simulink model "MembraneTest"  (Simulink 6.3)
settings: Solver=ode45  StartTime=0.0  StopTime=SimTime  FixedStep=0.001  RelTol=1e-3
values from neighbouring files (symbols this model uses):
  b = S/Sm    (= 0.1)    [Constantes.m]    (also in ConstantesBck.m)
  C = 1    [Constantes.m]    (also in ConstantesBck.m)
  Fact = 10^2    (= 100)    [Constantes.m]    (also in ConstantesBck.m)
  FreqStim = 1/(2*pi*i)    [SinPureTest.m]    (also in SinPureTestFreq.m; HalfSin.m; ScriptFour.m = 0.318309886184)
  gk = 36    [Constantes.m]    (also in ConstantesBck.m; sim_hh.m)
  gl = 0.3    [Constantes.m]    (also in ConstantesBck.m; sim_hh.m)
  gna = 120    [Constantes.m]    (also in ConstantesBck.m; sim_hh.m)
  h0 = 0.5961    [Constantes.m]    (also in ConstantesBck.m)
  IStim1 = AddI    (= 0)    [SinPureTest.m]    (also in SinPureTestFreq.m; ouin.m = -3000; TestStim.m; BiPhTest.m)
  m0 = 0.0529    [Constantes.m]    (also in ConstantesBck.m)
  mK = 0    [Constantes.m]    (also in ConstantesBck.m)
  mL = 0    [Constantes.m]    (also in ConstantesBck.m)
  mNa = 0    [Constantes.m]    (also in ConstantesBck.m)
  n0 = 0.3177    [Constantes.m]    (also in ConstantesBck.m)
  PhaseStim = 0    [SinPureTest.m]    (also in SinPureTestFreq.m; ScriptFour.m)
  Sm = 3.14e-2    (= 0.0314)    [Constantes.m]    (also in ConstantesBck.m = 0.000314)
  Vk = -82    [Constantes.m]    (also in ConstantesBck.m)
  Vl = -59    [Constantes.m]    (also in ConstantesBck.m)
  Vna = 45    [Constantes.m]    (also in ConstantesBck.m)
  Vr = -70    [Constantes.m]    (also in ConstantesBck.m)

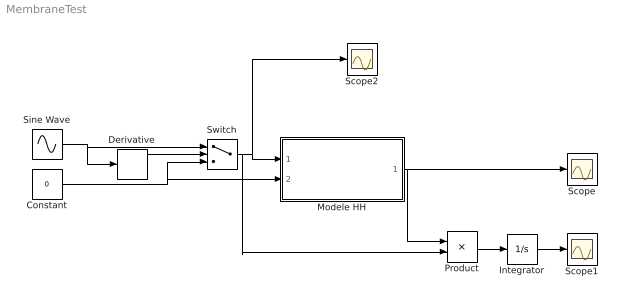
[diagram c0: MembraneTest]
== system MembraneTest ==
  Constant : Constant  Value=0
  Derivative : Derivative
  Integrator : Integrator
  Modele HH : Subsystem
  Product : Product
  Scope : Scope
  Scope1 : Scope
  Scope2 : Scope
  Sine Wave : Sin  Amplitude=IStim1  Frequency=FreqStim  Phase=PhaseStim  SampleTime=0
  Switch : Switch  Criteria=u2 > Threshold
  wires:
  Modele HH/1(HHout) -> Scope/1, Product/1
  Constant/1 -> Modele HH/2(VRefIn), Switch/3
  Sine Wave/1 -> Derivative/1, Switch/1
  Product/1 -> Integrator/1
  Integrator/1 -> Scope1/1
  Derivative/1 -> Switch/2
  Switch/1 -> Product/2, Modele HH/1(HHin), Scope2/1

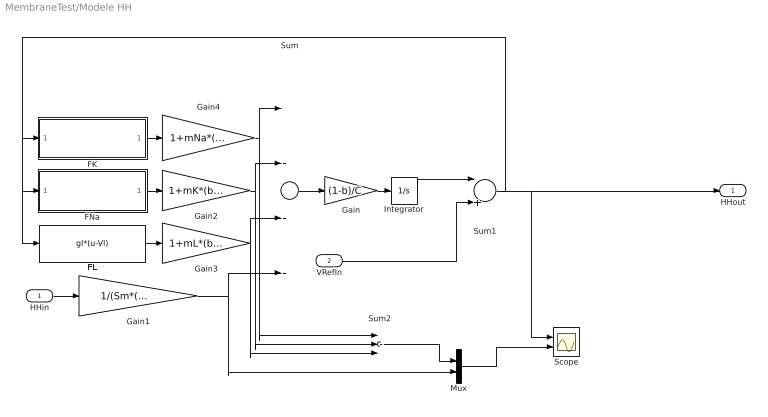
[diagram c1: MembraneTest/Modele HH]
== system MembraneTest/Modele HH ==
  HHin : Inport
  VRefIn : Inport  Port=2
  FK : Subsystem
  FL : Fcn  Expr=gl*(u-Vl)
  FNa : Subsystem
  Gain : Gain  Gain=(1-b)/C
  Gain1 : Gain  Gain=1/(Sm*(1-b)*Fact)
  Gain2 : Gain  Gain=1+mK*(b/(1-b))
  Gain3 : Gain  Gain=1+mL*(b/(1-b))
  Gain4 : Gain  Gain=1+mNa*(b/(1-b))
  Integrator : Integrator  InitialCondition=Vr
  Mux : Mux  Inputs=2
  Scope : Scope  NumInputPorts=2
  Sum : Sum  Inputs=|---+
  Sum1 : Sum  Inputs=|++
  Sum2 : Sum  Inputs=|+++
  HHout : Outport
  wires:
  Sum/1 -> Gain/1
  Gain/1 -> Integrator/1
  FK/1(FKout) -> Gain4/1
  FNa/1(FNaOut) -> Gain2/1
  FL/1 -> Gain3/1
  HHin/1 -> Gain1/1
  Integrator/1 -> Sum1/1
  Sum1/1 -> FNa/1(FNaIn), FL/1, FK/1(FKIn), HHout/1, Scope/1
  Gain1/1 -> Sum/4, Mux/2
  Gain4/1 -> Sum/1, Sum2/1
  Gain2/1 -> Sum/2, Sum2/2
  Gain3/1 -> Sum/3, Sum2/3
  VRefIn/1 -> Sum1/2
  Sum2/1 -> Mux/1
  Mux/1 -> Scope/2

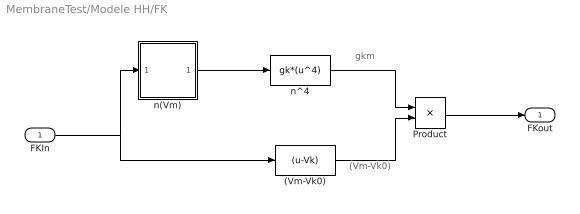
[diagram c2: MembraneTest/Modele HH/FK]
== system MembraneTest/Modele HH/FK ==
  note: gkm
  note: (Vm-Vk0)
  FKIn : Inport
  (Vm-Vk0) : Fcn  Expr=(u-Vk)
  Product : Product
  n(Vm) : Subsystem
  n^4 : Fcn  Expr=gk*(u^4)
  FKout : Outport  InitialOutput=0
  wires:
  n(Vm)/1(n) -> n^4/1
  (Vm-Vk0)/1 -> Product/2
  Product/1 -> FKout/1
  n^4/1 -> Product/1
  FKIn/1 -> n(Vm)/1(Vm), (Vm-Vk0)/1

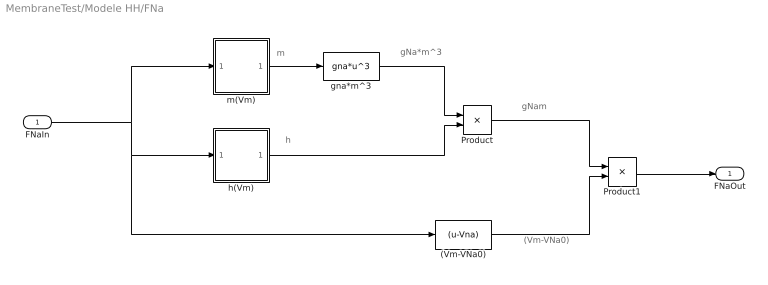
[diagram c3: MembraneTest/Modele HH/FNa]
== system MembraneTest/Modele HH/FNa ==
  note: gNa*m^3
  note: m
  note: h
  note: gNam
  note: (Vm-VNa0)
  FNaIn : Inport
  (Vm-VNa0) : Fcn  Expr=(u-Vna)
  Product : Product
  Product1 : Product
  gna*m^3 : Fcn  Expr=gna*u^3
  h(Vm) : Subsystem
  m(Vm) : Subsystem
  FNaOut : Outport  InitialOutput=0
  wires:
  (Vm-VNa0)/1 -> Product1/2
  gna*m^3/1 -> Product/1
  Product1/1 -> FNaOut/1
  FNaIn/1 -> m(Vm)/1(Vm), h(Vm)/1(Vm), (Vm-VNa0)/1
  m(Vm)/1(n) -> gna*m^3/1
  h(Vm)/1(h) -> Product/2
  Product/1 -> Product1/1

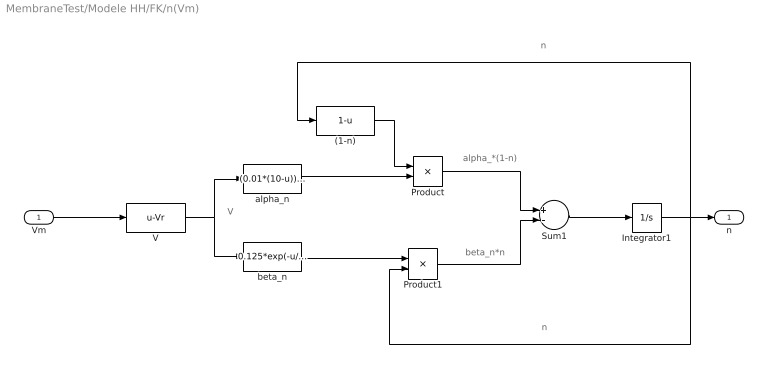
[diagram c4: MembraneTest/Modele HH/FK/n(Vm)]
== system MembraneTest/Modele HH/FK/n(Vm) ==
  note: V
  note: alpha_*(1-n)
  note: beta_n*n
  note: n
  note: n
  Vm : Inport
  (1-n) : Fcn  Expr=1-u
  Integrator1 : Integrator  InitialCondition=n0
  Product : Product
  Product1 : Product
  Sum1 : Sum  Inputs=+-
  V : Fcn  Expr=u-Vr
  alpha_n : Fcn  Expr=(0.01*(10-u))/(exp((10-u)/10)-1)
  beta_n : Fcn  Expr=0.125*exp(-u/80)
  n : Outport  InitialOutput=0
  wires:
  V/1 -> alpha_n/1, beta_n/1
  alpha_n/1 -> Product/2
  (1-n)/1 -> Product/1
  beta_n/1 -> Product1/1
  Product/1 -> Sum1/1
  Product1/1 -> Sum1/2
  Sum1/1 -> Integrator1/1
  Integrator1/1 -> (1-n)/1, Product1/2, n/1
  Vm/1 -> V/1

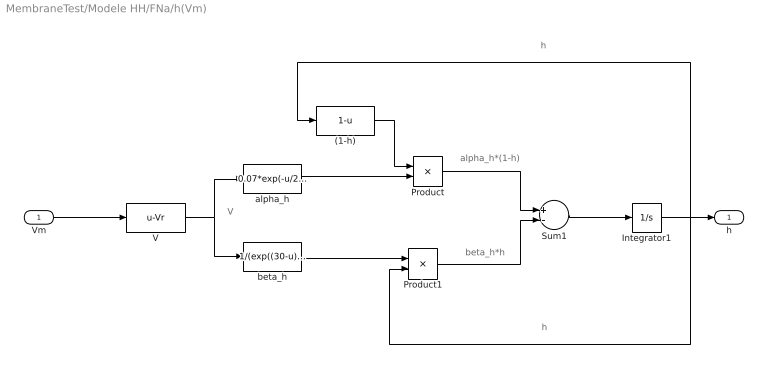
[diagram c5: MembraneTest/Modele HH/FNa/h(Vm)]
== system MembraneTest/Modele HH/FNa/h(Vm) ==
  note: h
  note: h
  note: beta_h*h
  note: alpha_h*(1-h)
  note: V
  Vm : Inport
  (1-h) : Fcn  Expr=1-u
  Integrator1 : Integrator  InitialCondition=h0
  Product : Product
  Product1 : Product
  Sum1 : Sum  Inputs=+-
  V : Fcn  Expr=u-Vr
  alpha_h : Fcn  Expr=0.07*exp(-u/20)
  beta_h : Fcn  Expr=1/(exp((30-u)/10)+1)
  h : Outport  InitialOutput=0
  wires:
  Vm/1 -> V/1
  Integrator1/1 -> h/1, Product1/2, (1-h)/1
  Sum1/1 -> Integrator1/1
  Product1/1 -> Sum1/2
  Product/1 -> Sum1/1
  beta_h/1 -> Product1/1
  (1-h)/1 -> Product/1
  alpha_h/1 -> Product/2
  V/1 -> beta_h/1, alpha_h/1

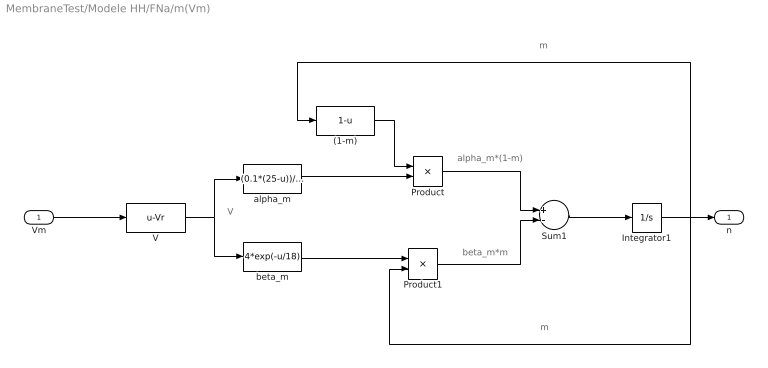
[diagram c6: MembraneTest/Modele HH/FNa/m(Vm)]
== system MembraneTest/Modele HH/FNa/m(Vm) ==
  note: m
  note: m
  note: beta_m*m
  note: alpha_m*(1-m)
  note: V
  Vm : Inport
  (1-m) : Fcn  Expr=1-u
  Integrator1 : Integrator  InitialCondition=m0
  Product : Product
  Product1 : Product
  Sum1 : Sum  Inputs=+-
  V : Fcn  Expr=u-Vr
  alpha_m : Fcn  Expr=(0.1*(25-u))/(exp((25-u)/10)-1)
  beta_m : Fcn  Expr=4*exp(-u/18)
  n : Outport  InitialOutput=0
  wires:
  Vm/1 -> V/1
  Integrator1/1 -> n/1, Product1/2, (1-m)/1
  Sum1/1 -> Integrator1/1
  Product1/1 -> Sum1/2
  Product/1 -> Sum1/1
  beta_m/1 -> Product1/1
  (1-m)/1 -> Product/1
  alpha_m/1 -> Product/2
  V/1 -> beta_m/1, alpha_m/1
